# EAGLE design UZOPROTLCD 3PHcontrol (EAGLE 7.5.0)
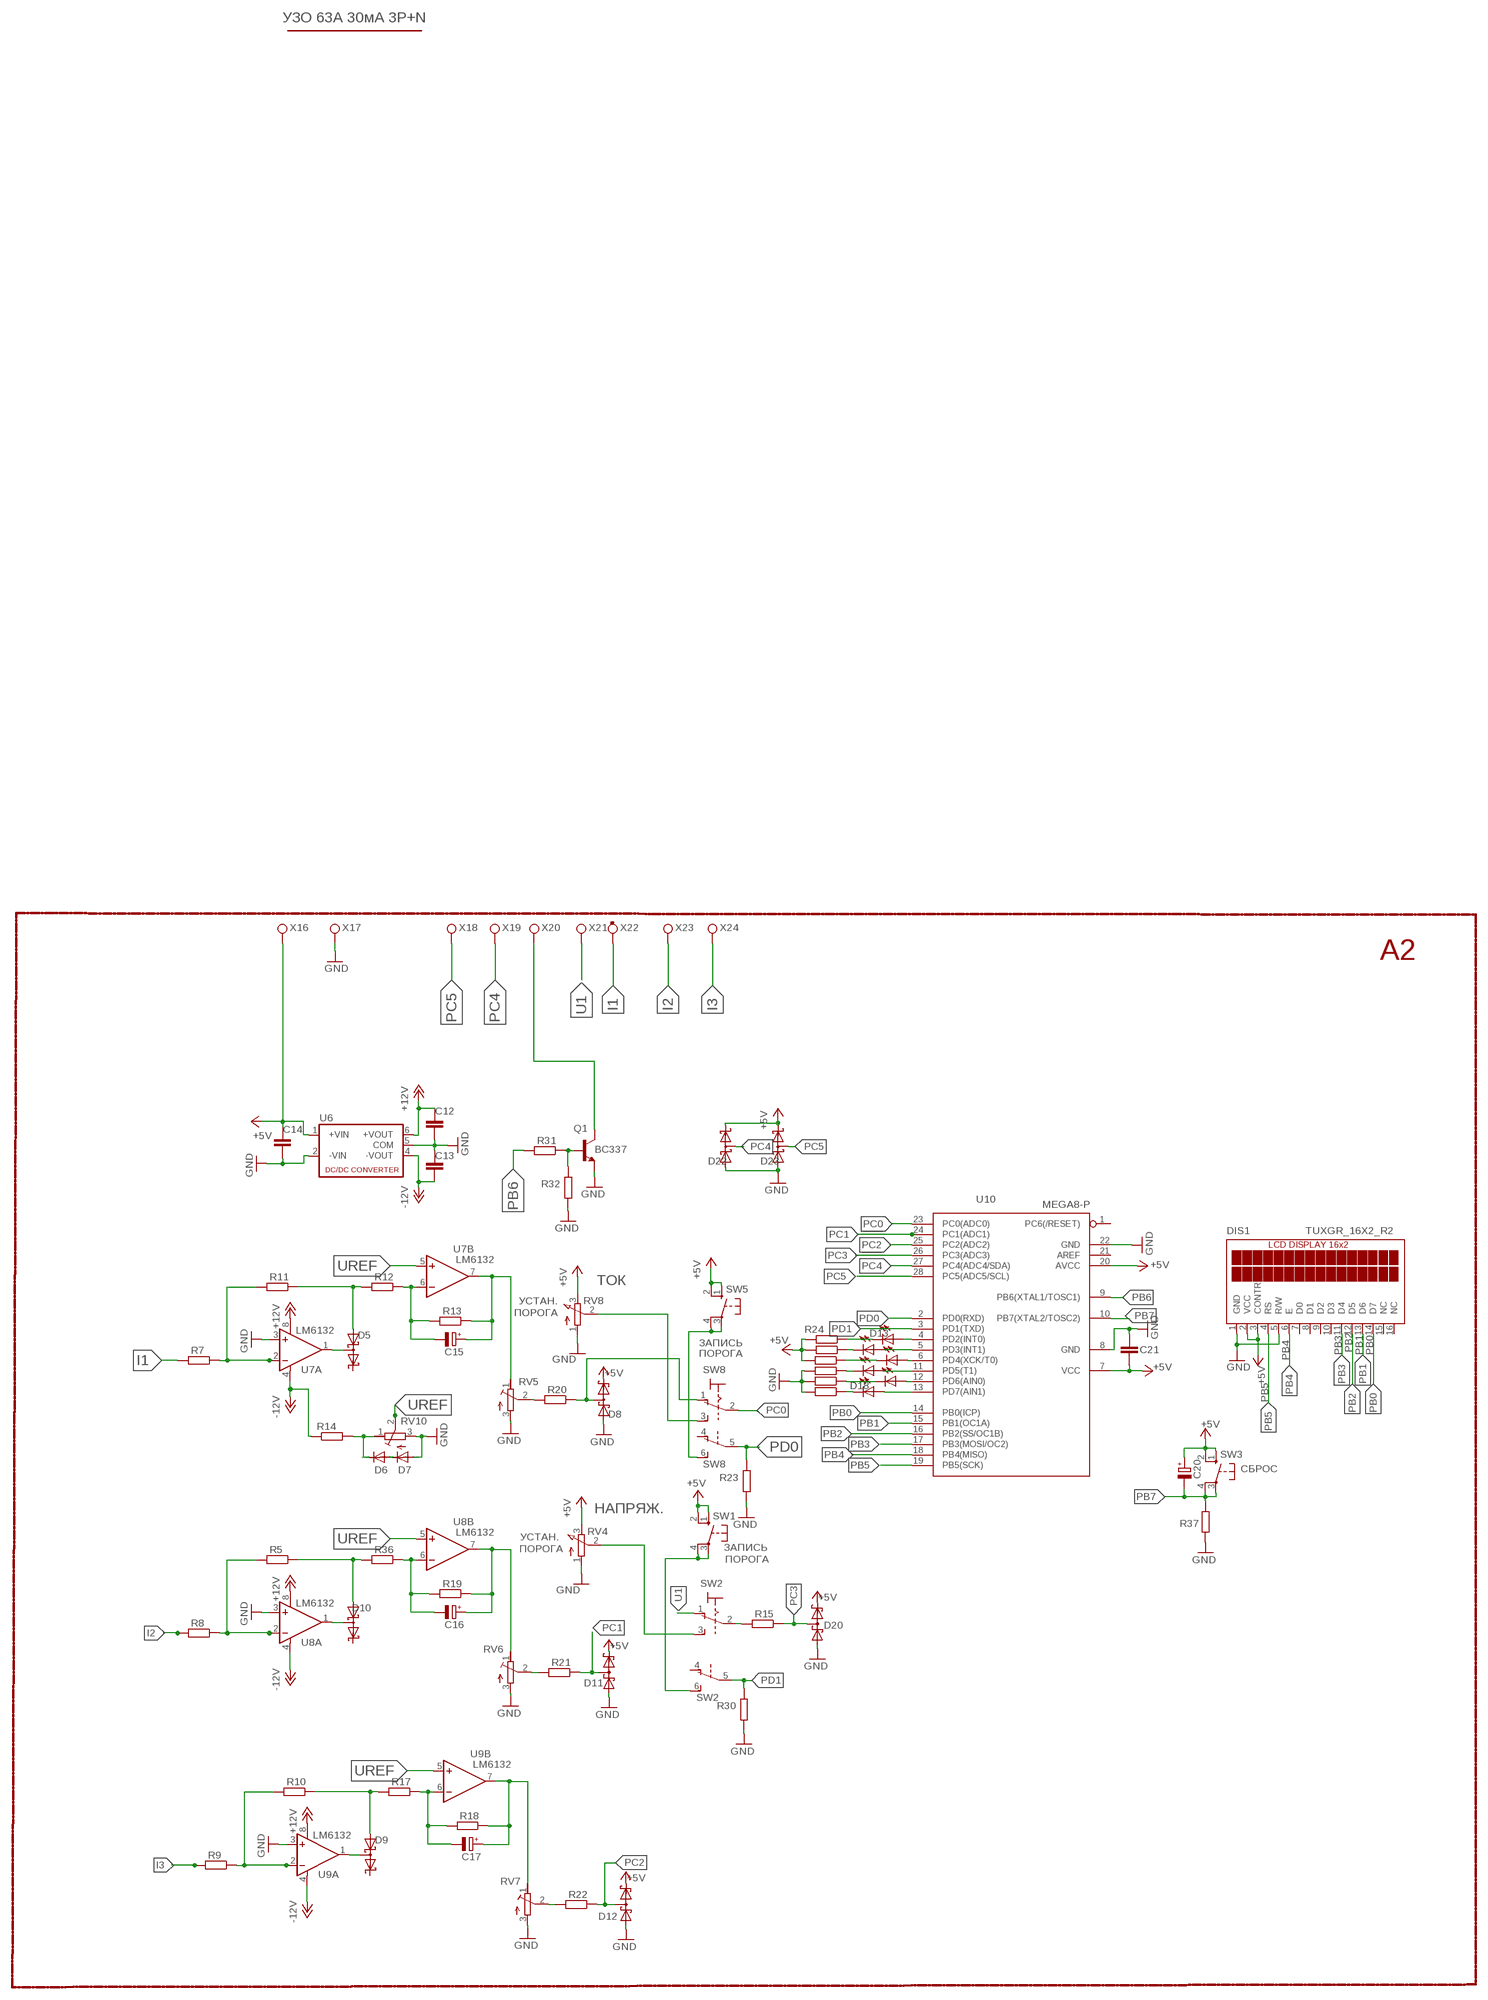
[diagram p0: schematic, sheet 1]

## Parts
C12  C-EUC1206  [C1206]
C13  C-EUC1206  [C1206]
C14  C-EUC1206  [C1206]
C15  CPOL-EUE2-4  [E2-4]
C16  CPOL-EUE2-4  [E2-4]
C17  CPOL-EUE2-4  [E2-4]
C20  CPOL-EUE2-5  [E2-5]
C21  C-EUC1206  [C1206]
D5  BAT54S  [SOT23]
D6  1N4148DO35-7  [DO35-7]
D7  1N4148DO35-7  [DO35-7]
D8  BAT54S  [SOT23]
D9  BAT54S  [SOT23]
D10  BAT54S  [SOT23]
D11  BAT54S  [SOT23]
D12  BAT54S  [SOT23]
D13  LED3MM  [LED3MM]
D14  LED3MM  [LED3MM]
D15  LED3MM  [LED3MM]
D16  LED3MM  [LED3MM]
D17  LED3MM  [LED3MM]
D18  LED3MM  [LED3MM]
D20  BAT54S  [SOT23]
D22  BAT54S  [SOT23]
D23  BAT54S  [SOT23]
DIS1  TUXGR_16X2_R2  [TUXGR_16X2_R2]
Q1  BC337  [TO92]
R5  R-EU_R1206  [R1206]
R7  R-EU_R1206  [R1206]
R8  R-EU_R1206  [R1206]
R9  R-EU_R1206  [R1206]
R10  R-EU_R1206  [R1206]
R11  R-EU_R1206  [R1206]
R12  R-EU_R1206  [R1206]
R13  R-EU_R1206  [R1206]
R14  R-EU_R1206  [R1206]
R15  R-EU_R1206  [R1206]
R17  R-EU_R1206  [R1206]
R18  R-EU_R1206  [R1206]
R19  R-EU_R1206  [R1206]
R20  R-EU_R1206  [R1206]
R21  R-EU_R1206  [R1206]
R22  R-EU_R1206  [R1206]
R23  R-EU_R1206  [R1206]
R24  R-EU_R1206  [R1206]
R25  R-EU_R1206  [R1206]
R26  R-EU_R1206  [R1206]
R27  R-EU_R1206  [R1206]
R28  R-EU_R1206  [R1206]
R29  R-EU_R1206  [R1206]
R30  R-EU_R1206  [R1206]
R31  R-EU_R1206  [R1206]
R32  R-EU_R1206  [R1206]
R36  R-EU_R1206  [R1206]
R37  R-EU_R1206  [R1206]
RV4  PTV09A  PV09A  [PTV09]
RV5  R-TRIMM-3386-F  [R-TRIMM-3386F]
RV6  R-TRIMM-3386-F  [R-TRIMM-3386F]
RV7  R-TRIMM-3386-F  [R-TRIMM-3386F]
RV8  PTV09A  PV09A  [PTV09]
RV10  R-TRIMM-3386-F  [R-TRIMM-3386F]
SW1  SPST Push Button  10-XX  [B3F-10XX]
SW2  320-938  [320-938]
SW3  SPST Push Button  10-XX  [B3F-10XX]
SW5  SPST Push Button  10-XX  [B3F-10XX]
SW8  320-938  [320-938]
U6  NMA  [NMA]
U7  LM6132  OPA2134P  [DIL08]
U8  LM6132  OPA2134P  [DIL08]
U9  LM6132  OPA2134P  [DIL08]
U10  MEGA8-P  [DIL28-3]
X16  TPPAD1-17  [P1-17]
X17  TPPAD1-17  [P1-17]
X18  TPPAD1-17  [P1-17]
X19  TPPAD1-17  [P1-17]
X20  TPPAD1-17  [P1-17]
X21  TPPAD1-17  [P1-17]
X22  TPPAD1-17  [P1-17]
X23  TPPAD1-17  [P1-17]
X24  TPPAD1-17  [P1-17]

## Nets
+5V: C14.1 C20.+ C21.2 D8.2(C2) D11.2(C2) D12.2(C2) D20.2(C2) D22.2(C2) D23.2(C2) DIS1.2(VCC) DIS1.3(CONTR) R24.2 R25.2 R26.2 RV4.3(E) RV8.3(E) SW1.1(S) SW1.2(S1) SW3.1(S) SW3.2(S1) SW5.1(S) SW5.2(S1) U6.1(+VIN) U10.7(VCC) U10.20(AVCC) X16.TP
+12V: C12.1 U6.6(+VOUT) U7.8(A:V+) U8.8(A:V+) U9.8(A:V+)
-12V: C13.2 R14.1 U6.4(-VOUT) U7.4(A:V-) U8.4(A:V-) U9.4(A:V-)
GND: C12.2 C13.1 C14.2 C21.1 D7.A D8.1(A1) D11.1(A1) D12.1(A1) D20.1(A1) D22.1(A1) D23.1(A1) DIS1.1(GND) DIS1.5(R/W) Q1.1(E) R23.2 R27.2 R28.2 R29.2 R30.2 R32.2 R37.2 RV4.1(A) RV5.3(E) RV6.3(E) RV7.3(E) RV8.1(A) RV10.3(E) U6.2(-VIN) U6.5(COM) U7.3(A:+IN) U8.3(A:+IN) U9.3(A:+IN) U10.8(GND) U10.22(GND) X17.TP
I1: R7.2 X22.TP
I2: R8.2 X23.TP
I3: R9.2 X24.TP
N$40: Q1.2(B) R31.1 R32.1
N$41: R7.1 R11.2 U7.2(A:-IN)
N$42: Q1.3(C) X20.TP
N$43: D6.C R14.2 RV10.1(A)
N$44: D6.A D7.C
N$45: D5.1(A1) R11.1 R12.2
N$46: D5.3(C1A2) U7.1(A:OUT)
N$47: C15.- R12.1 R13.2 U7.6(B:-IN)
N$48: C15.+ R13.1 RV5.1(A) U7.7(B:OUT)
N$49: R20.2 RV5.2(S)
N$50: RV8.2(S) SW8.3(1:S)
N$51: SW5.3(P) SW5.4(P1) SW8.6(B:S)
N$52: D8.3(C1A2) R20.1 SW8.1(1:O)
N$53: R9.1 R10.2 U9.2(A:-IN)
N$54: R5.2 R8.1 U8.2(A:-IN)
N$55: D10.1(A1) R5.1 R36.2
N$56: D10.3(C1A2) U8.1(A:OUT)
N$57: C16.- R19.2 R36.1 U8.6(B:-IN)
N$58: C16.+ R19.1 RV6.1(A) U8.7(B:OUT)
N$59: R21.2 RV6.2(S)
N$60: D9.1(A1) R10.1 R17.2
N$61: D9.3(C1A2) U9.1(A:OUT)
N$62: C17.- R17.1 R18.2 U9.6(B:-IN)
N$63: C17.+ R18.1 RV7.1(A) U9.7(B:OUT)
N$64: R22.2 RV7.2(S)
N$65: RV4.2(S) SW2.3(1:S)
N$66: SW1.3(P) SW1.4(P1) SW2.6(B:S)
N$67: R15.2 SW2.2(1:P)
N$68: D13.A U10.4(PD2(INT0))
N$69: D13.K(C) R24.1
N$70: D14.A U10.5(PD3(INT1))
N$71: D14.K(C) R25.1
N$72: D15.K(C) R26.1
N$74: D16.K(C) R27.1
N$75: D17.K(C) R28.1
N$76: D18.K(C) R29.1
N$77: D15.A U10.6(PD4(XCK/T0))
N$78: D16.A U10.11(PD5(T1))
N$79: D17.A U10.12(PD6(AIN0))
N$80: D18.A U10.13(PD7(AIN1))
PB0: DIS1.14(D7) U10.14(PB0(ICP))
PB1: DIS1.13(D6) U10.15(PB1(OC1A))
PB2: DIS1.12(D5) U10.16(PB2(SS/OC1B))
PB3: DIS1.11(D4) U10.17(PB3(MOSI/OC2))
PB4: DIS1.6(E) U10.18(PB4(MISO))
PB5: DIS1.4(RS) U10.19(PB5(SCK))
PB6: R31.2 U10.9(PB6(XTAL1/TOSC1))
PB7: C20.- R37.1 SW3.3(P) SW3.4(P1) U10.10(PB7(XTAL2/TOSC2))
PC0: SW8.2(1:P) U10.23(PC0(ADC0))
PC1: D11.3(C1A2) R21.1 U10.24(PC1(ADC1))
PC2: D12.3(C1A2) R22.1 U10.25(PC2(ADC2))
PC3: D20.3(C1A2) R15.1 U10.26(PC3(ADC3))
PC4: D22.3(C1A2) U10.27(PC4(ADC4/SDA)) X19.TP
PC5: D23.3(C1A2) U10.28(PC5(ADC5/SCL)) X18.TP
PD0: R23.1 SW8.5(B:P) U10.2(PD0(RXD))
PD1: R30.1 SW2.5(B:P) U10.3(PD1(TXD))
U1: SW2.1(1:O) X21.TP
UREF: RV10.2(S) U7.5(B:+IN) U8.5(B:+IN) U9.5(B:+IN)
Unconnected: D5.2(C2) D9.2(C2) D10.2(C2) DIS1.7(D0) DIS1.8(D1) DIS1.9(D2) DIS1.10(D3) DIS1.15(NC) DIS1.16(NC) SW2.4(B:O) SW8.4(B:O) U10.1(PC6(/RESET)) U10.21(AREF)

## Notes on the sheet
- УЗО 63А 30мА 3Р+N
- A2
- ТОК
- УСТАН.
- ПОРОГА
- ЗАПИСЬ
- ПОРОГА
- СБРОС
- НАПРЯЖ.
- УСТАН.
- ПОРОГА | ЗАПИСЬ
- ПОРОГА

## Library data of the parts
C12-C14 C21 = rcl:C-EU: CAPACITOR, European symbol
C15-C17 C20 = rcl:CPOL-EU: POLARIZED CAPACITOR, European symbol
D5 D8-D12 D20 D22 D23 = diode:BAT54S: Schottky Diodes Pin connection corrected 2011-05-04 Source: Fairchild .. BAT54.pdf
D6 D7 = diode:1N4148: DIODE
D13-D18 = led:LED: LED
DIS1 = display-lcd:TUXGR_16X2_R2: Tuxgraphics LCD display 16x2 characters reflective, without background light Source: tuxgr_12x2_r2.pdf; OC_FARNELL: unknown; OC_NEWARK: unknown
Q1 = transistor:BC337: NPN TRANSISTOR
R5 R7-R15 R17-R32 R36 R37 = rcl:R-EU_: RESISTOR, European symbol
RV4 RV8 = pot:PV09A
RV5-RV7 RV10 = rcl:R-TRIMM-3386-F
SW1 SW3 SW5 = switch-omron:10-XX: OMRON SWITCH; MPN: B3F-1000; OC_FARNELL: 176432; OC_NEWARK: 36M3542
SW2 SW8 = switch:320-938: TOGGLE SWITCH distributor RS Components
U6 = dc-dc-converter:NMA: DC-DC CONVERTER; MF: C & D TECHNOLOGIES, INC; MPN: NMA0515SC; OC_FARNELL: 1021434; OC_NEWARK: 61K3064
U7-U9 = burr-brown:OPA2134: Operational Amplifier; MF: TEXAS INSTRUMENTS; MPN: OPA2134PA; OC_FARNELL: 1097574; OC_NEWARK: 74K3897
U10 = atmel:MEGA8-P: MICROCONTROLLER 8 Kbytes FLASH, 1 kbytes SRAM, 512 bytes EEPROM, USART, 4-channel 10 bit ADC, 2-channel 8 bit ADC Pin compatible with Atmega48, ATMega88, ATMega168 Source: avr.lbr; OC_FARNELL: unknown; OC_NEWARK: unknown
X16-X24 = testpad:TP: Test pad

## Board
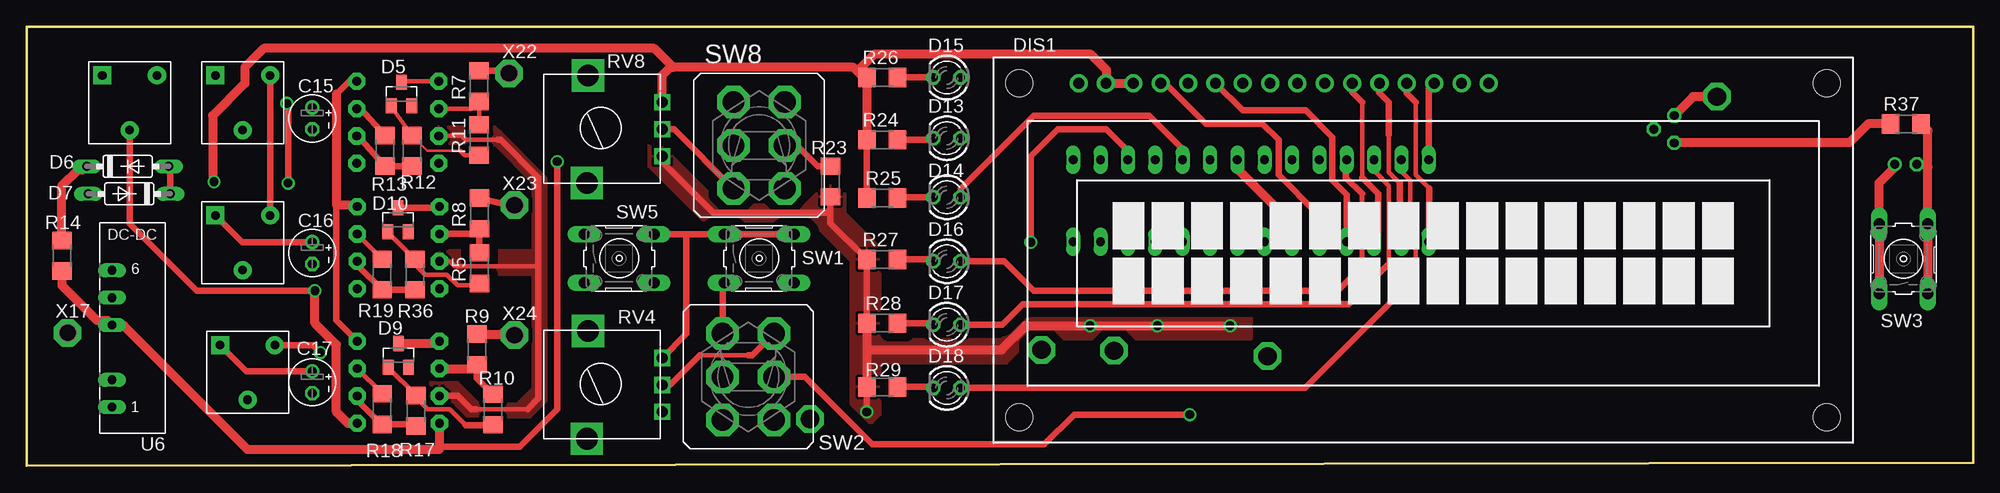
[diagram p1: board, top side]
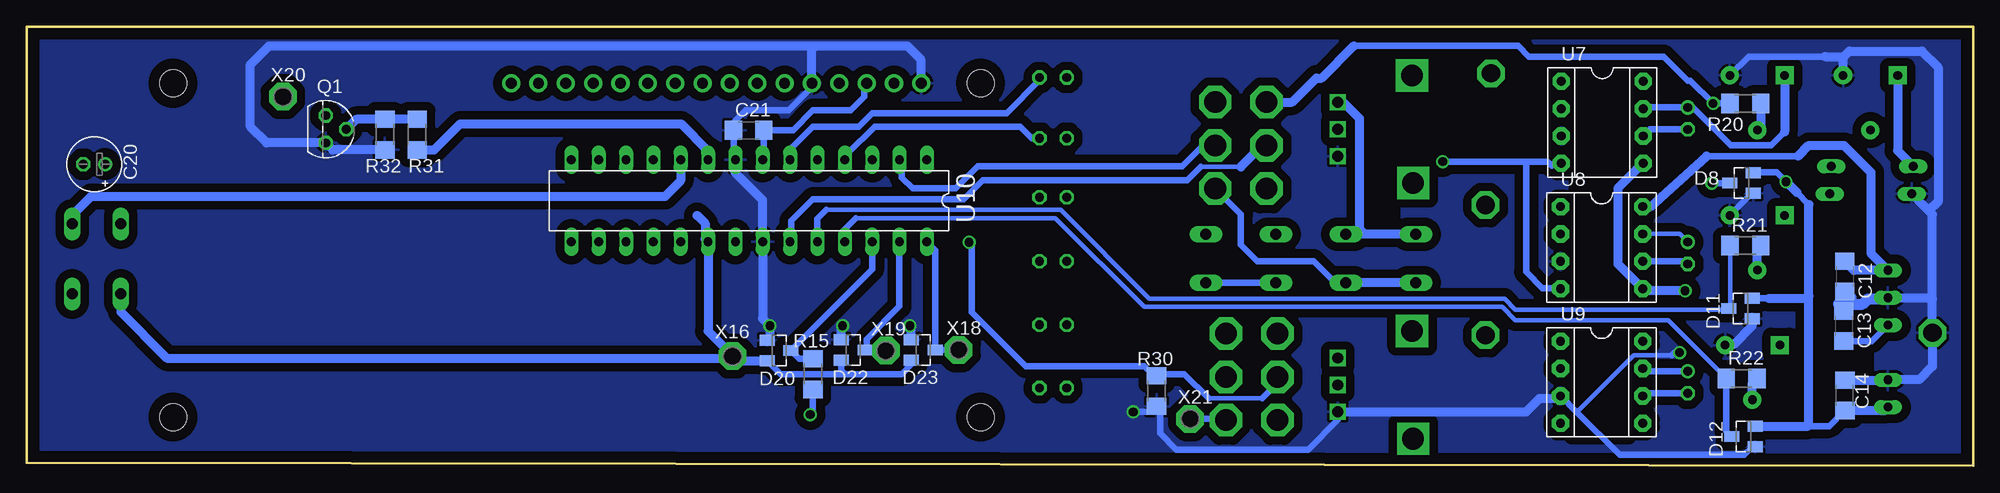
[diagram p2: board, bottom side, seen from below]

Size 180.75 x 40.75 mm. Coordinates in mm from the lower left corner, seen from the top.
Outline: 0,0 180.75,0.25 180.75,40.75 0,40.75 0,0
Copper layers (1*16): Top 0.035mm / dielectric 1.5mm / Bottom 0.035mm
Design rules "default": minimum track width 10mil, minimum drill 24mil, track to track 8mil, track to pad 8mil, pad to pad 8mil, via to via 8mil, smd to smd 8mil, copper to edge 40mil, drill to drill 8mil, minimum pad ring 10mil, minimum via ring 8mil, stop-mask expansion 4mil, vias tented up to drill 0mil, thermal gap 10mil
bRestrict: area 10,4.8 to 14.5,24.5; area 10.5,23.8 to 12.5,24; area 31.8,15.2 to 36.8,37; area 32,2.8 to 37.2,12.8; area 39.2,29.2 to 55.5,37; area 54,23 to 55.8,28.8

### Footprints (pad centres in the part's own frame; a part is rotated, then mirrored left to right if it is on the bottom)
C1206 = smd 1.6 x 1.8: 1 -1.4,0; 2 1.4,0
E2-4 = drill 0.813 pad 1.27: + -1.016,0 | drill 0.813 pad 1.27 octagon: - 1.016,0
E2-5 = drill 0.813 pad 1.27: + -1.016,0 | drill 0.813 pad 1.27 octagon: - 1.016,0
SOT23 = smd 1 x 1.4: 1 -0.95,-1.1; 2 0.95,-1.1; 3 0,1.1
DO35-7 = drill 0.813 long: A 3.81,0; C -3.81,0
LED3MM = drill 0.813 octagon: A -1.27,0; K 1.27,0
TUXGR_16X2_R2 = drill 1 pad 1.676: 1 -32,15.5; 2 -29.46,15.5; 3 -26.92,15.5; 4 -24.38,15.5; 5 -21.84,15.5; 6 -19.3,15.5; 7 -16.76,15.5; 8 -14.22,15.5; 9 -11.68,15.5; 10 -9.14,15.5; 11 -6.6,15.5; 12 -4.06,15.5; 13 -1.52,15.5; 14 1.02,15.5; 15 3.56,15.5; 16 6.1,15.5 | hole 2.5: -37.5,-15.5; 37.5,-15.5; -37.5,15.5; 37.5,15.5
TO92 = drill 0.813 octagon: 1 1.27,0; 2 0,1.905; 3 -1.27,0
R1206 = smd 1.6 x 1.803: 1 -1.422,0; 2 1.422,0
PTV09 = drill 1 square: 1 -2.5,0; 2 0,0; 3 2.5,0 | drill 2 square: P$4 -5,7; P$5 5,6.9
R-TRIMM-3386F = drill 0.8 pad 1.676 square: 1 0,0 | drill 0.8 pad 1.676: 2 5.08,2.54; 3 0,5.08
B3F-10XX = drill 1.016 long: 1 -3.251,2.261; 2 3.251,2.261; 3 -3.251,-2.261; 4 3.251,-2.261
320-938 = drill 2.007 octagon: 1 -2.388,4.013; 2 -2.388,0; 3 -2.388,-4.013; 4 2.388,4.013; 5 2.388,0; 6 2.388,-4.013
NMA = drill 0.813 long: 1 0,6.35; 2 0,3.81; 4 0,-1.27; 5 0,-3.81; 6 0,-6.35
DIL08 = drill 0.813 pad 1.6 octagon: 1 -3.81,-3.81; 2 -1.27,-3.81; 3 1.27,-3.81; 4 3.81,-3.81; 5 3.81,3.81; 6 1.27,3.81; 7 -1.27,3.81; 8 -3.81,3.81
DIL28-3 = drill 0.813 long: 1 -16.51,-3.81; 2 -13.97,-3.81; 3 -11.43,-3.81; 4 -8.89,-3.81; 5 -6.35,-3.81; 6 -3.81,-3.81; 7 -1.27,-3.81; 8 1.27,-3.81; 9 3.81,-3.81; 10 6.35,-3.81; 11 8.89,-3.81; 12 11.43,-3.81; 13 13.97,-3.81; 14 16.51,-3.81; 15 16.51,3.81; 16 13.97,3.81; 17 11.43,3.81; 18 8.89,3.81; 19 6.35,3.81; 20 3.81,3.81; 21 1.27,3.81; 22 -1.27,3.81; 23 -3.81,3.81; 24 -6.35,3.81; 25 -8.89,3.81; 26 -11.43,3.81; 27 -13.97,3.81; 28 -16.51,3.81
P1-17 = drill 1.702 pad 2.54 octagon: TP 0,0

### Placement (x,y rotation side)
C12  11.92,17.58 270 bottom
C13  12.01,12.97 270 bottom
C14  11.91,6.53 90 bottom
C15  26.5,32.25 270 top
C16  26.5,19.75 270 top
C17  26.5,7.75 270 top
C20  174.5,28 180 bottom
C21  113.72,31.15 0 bottom
D5  34.78,34.52 0 top
D6  9.36,27.8 0 top
D7  9.5,25.25 180 top
D8  21.5,26.25 90 bottom
D9  34.5,10.25 0 top
D10  34.47,22.84 0 top
D11  21.61,14.6 90 bottom
D12  21.33,2.72 90 bottom
D13  85.44,30.42 180 top
D14  85.44,24.93 180 top
D15  85.44,36.05 180 top
D16  85.44,18.98 180 top
D17  85.44,13.1 180 top
D18  85.44,7.22 180 top
D20  110.89,10.69 270 bottom
D22  104,10.75 270 bottom
D23  97.5,10.75 270 bottom
DIS1  129.68,20.02 0 top
Q1  153,31.25 270 bottom
R5  42.03,18.35 90 top
R7  42,35.25 90 top
R8  42.03,23.43 90 top
R9  41.79,10.8 90 top
R10  43.29,5.22 90 top
R11  42,30.25 90 top
R12  35.75,29.25 90 top
R13  33.25,29.25 270 top
R14  3.25,19.5 90 top
R15  107.75,8.5 270 bottom
R17  36.14,5.1 90 top
R18  33,5.25 270 top
R19  33,17.75 270 top
R20  21.15,33.64 0 bottom
R21  21.15,20.44 0 bottom
R22  21.49,8.11 0 bottom
R23  74.63,26.4 270 top
R24  79.44,30.27 180 top
R25  79.44,24.85 180 top
R26  79.44,36.07 180 top
R27  79.44,19.15 180 top
R28  79.44,13.23 180 top
R29  79.44,7.31 180 top
R30  75.84,6.94 270 bottom
R31  144.5,30.75 270 bottom
R32  147.5,30.75 270 bottom
R36  36.03,17.76 90 top
R37  174.5,31.75 180 top
RV4  59,7.5 90 top
RV5  17.5,36.25 270 top
RV6  17.5,23.25 270 top
RV7  17.95,11.2 270 top
RV8  59,31.25 90 top
RV10  7,36.25 270 top
SW1  68,19.25 0 top
SW2  67,8.25 180 top
SW3  174.29,19.21 90 top
SW5  55,19.25 0 top
SW8  68,29.75 0 top
U6  7.91,11.79 180 top
U7  34.44,31.89 270 bottom
U8  34.5,20.25 270 bottom
U9  34.5,7.75 270 bottom
U10  113.68,24.61 180 bottom
X16  115.22,10.17 0 bottom
X17  3.78,12.34 0 top
X18  94.22,10.76 0 bottom
X19  100.97,10.68 0 bottom
X20  156.97,34.27 0 bottom
X21  72.72,4.35 0 bottom
X22  44.78,36.44 0 top
X23  45.28,24.2 0 top
X24  45.28,12.12 0 top

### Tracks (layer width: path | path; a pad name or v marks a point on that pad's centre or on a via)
+5V  (via drill 0.8)
  Top 0.61: R25.2 R24.2 | SW5.2 61.25,21.51 | 61.25,21.51 SW1.1 SW1.2 | RV4.3 61.25,12.25 61.25,21.51
  Top 0.813: 77.12,36.62 77.68,36.07 R26.2 R24.2 | 77.12,36.62 76.75,37 60,37 59.88,37.12 | U10.7 112.41,27.59 117.25,22.75 117.25,21.04 U10.20 | C20.+ 173.48,27.73 172,26.25 172,22.49 SW3.2 SW3.1 | 77.12,36.62 78.75,38.25 98.75,38.25 100.25,36.75 100.25,35.55 DIS1.2 DIS1.3 | 59.88,37.12 58.25,38.75 22,38.75 20.25,37 20.25,35.5 17.25,32.5 17.25,26.5 v17.38,26.38 | RV8.3 59,36.25 59.88,37.12
  Bottom 0.61: U10.7 112.32,28.51 C21.2 109.6,31.15 107.75,33 104.25,33 103,34.25 103,35.28 DIS1.3 | D23.2 98.6,9.4 99.5,8.5 104.75,8.5 | 104.75,8.5 110.75,8.5 | 110.75,8.5 D20.2 | D22.2 105.1,8.85 104.75,8.5 | 110.72,8.47 110.75,8.5 | D20.2 114.8,9.75 X16.TP | D11.2 18.95,15.55 | D12.2 13.37,3.67 C14.1 | 15.25,24.25 16.38,25.38 | v17.38,26.38 18.25,27.25 20.35,27.25 D8.2
  Bottom 0.813: D20.2 114.75,9.75 117.49,12.49 U10.20 117.75,21.06 117.75,22.5 118.5,23.25 | SW3.1 172.03,14.28 167.75,10 115.05,10 114.8,9.75 | RV8.3 58.5,33.75 57,32.25 57,22.01 56.5,21.51 | SW5.1 56.5,21.51 | 56.5,21.51 SW5.2 | C14.1 8.22,5.13 U6.1 | D12.2 15.33,3.67 15.25,3.75 15.25,15.75 | 18.95,15.55 15.45,15.55 15.25,15.75 | 15.25,15.75 15.25,24.25 | v17.38,26.38 16.38,25.38
+12V
  Top 0.61: U7.8 29.95,35.7 28.75,34.5 | 28.75,24.25 28.75,13.5 U9.8
  Top 0.813: 28.75,34.5 28.75,24.25 30.5,24.25 U8.8
  Bottom 0.61: 24.75,28.75 16.25,28.75
  Bottom 0.813: C12.1 11.08,18.14 U6.6 9.5,19.73 9.5,27.25 12,29.75 15.25,29.75 16.25,28.75 | U8.8 29.94,24.06 24.75,28.75
-12V  (via drill 0.8)
  Top 0.61: 38.31,1.75 45.75,1.75 49.25,5.25 v49.25,28.25
  Top 0.813: U9.4 38.31,1.75 38.31,1.56 38.25,1.5 20.5,1.5 9,13 7.97,13 U6.4 7.47,13.5 6.5,13.5 3.25,16.75 R14.1
  Bottom 0.61: U7.4 38.92,28.08 39.12,27.88 39.5,28.25 41.5,28.25 | 41.5,28.25 41.5,18 40,16.5 38.37,16.5 U8.4 | v49.25,28.25 41.5,28.25 | C13.2 9.4,11.57 U6.4
GND  (via drill 0.8)
  Top 0.406: U7.3 40.38,30.62 40.75,30.25 43.75,30.25 | 47.5,18.5 39.75,18.5 39.25,19 38.33,19 U8.3 | 46.5,5.25 41.75,5.25
  Top 0.61: R23.2 74.63,23.75 | 74.63,23.75 74.63,22.54 R27.2 R28.2 78.02,10.77 78,10.75 | RV8.1 59,28.25 63.75,23.5 74.38,23.5 74.63,23.75 | R29.2 78.02,5.02 v78,5 | 43.75,30.25 44,30.25 47.5,26.75 47.5,18.5 47.5,6.25 46.5,5.25 | 41.75,5.25 41.25,5.25 40,6.5 38.33,6.5 U9.3 | RV6.3 RV5.3 | v27.25,10.5 26.55,11.2 RV7.3
  Top 0.813: v111.75,13 v105,13 v98.75,13 92.75,13 90.5,10.75 78,10.75 | R28.2 R29.2 | R37.2 171,31.75 169.25,30 153.02,30 Q1.1
  Bottom 0.305: 11.75,14.5 11.5,14.5 11,15
  Bottom 0.406: 28,10.25 31.5,10.25 36.79,4.96
  Bottom 0.61: U10.8 115.12,28.59 C21.1 115,31.27 115,32 114,33 110,33 107.84,35.16 DIS1.5 | RV4.1 59,4.25 61.75,1.5 74,1.5 75.5,3 75.5,5.18 R30.2 76.36,5 v78,5 | RV10.3 12.08,36.33 | 13.75,38 20.83,38 RV5.3 | RV7.3 22.96,11.2 | D8.1 20.4,25.43 RV6.3 | D12.1 20.48,1.77 21.25,1 32.83,1 36.79,4.96 U9.3 | v27.25,10.5 27.75,10.5 28,10.25
  Bottom 0.813: D20.1 111.75,11.88 v111.75,13 112.41,13.66 U10.22 112.41,24.66 115,27.25 115,28.37 U10.8 | D22.1 105.1,12.9 v105,13 | D23.1 98.6,12.85 v98.75,13 | R32.2 152.35,29.33 Q1.1 158.48,29.98 160,31.5 160,37.25 158.25,39 107.5,39 | 107.5,39 99,39 97.75,37.75 97.75,35.59 DIS1.1 | DIS1.5 107.84,38.66 107.5,39 | RV4.1 41.5,5 40.25,6.25 38.54,6.25 U9.3 | 12.01,16.09 C12.2 11.34,15.6 | 12.14,14.5 C13.1 11.88,14.37 11.75,14.5 | 3.78,15.5 X17.TP 3.78,9.22 5,8 7.89,8 U6.2 7.96,7.93 C14.2 | 3.78,15.5 3.78,23.34 4.09,23.66 | 4.09,23.66 D7.A | U6.5 3.88,15.6 3.78,15.5 | D11.1 20.51,12.99 22.25,11.25 22.91,11.25 22.96,11.2 | 13.75,38 12,38 | 12,38 11.5,38.5 4.75,38.5 3.25,37 3.25,24.5 4.09,23.66 | 12.08,36.33 12.08,37.92 12,38
  Bottom 1.016: 11.34,15.6 11.9,15.6 12.5,15 11,15 10.25,15 9.75,15.5 8.01,15.5 U6.5
  pour Bottom (isolate 0.8): 1,39.75 180,39.5 180,1 1,1.25
  pour Top (isolate 0.406): 44,31 48.25,26.75 48.25,6 46.75,4.5 38.5,4.5 37.25,5.75 37.25,7.5 37.5,7.75 40,7.75 42,5.75 45.5,5.75 47,7.25 47,26.25 43.5,29.75 37.75,29.75 37.5,30 37.5,31.25 37.75,31.5 43.5,31.5
  pour Top (isolate 0.813): 58.25,30 58.75,30 64.5,24.25 72.25,24.25 74,26 75.25,26 76,25.25 76,23.5 79.25,20.25 79.25,4.75 78.5,4 77.5,4 76.75,4.75 76.5,5 76.5,19 73,22.5 63,22.5 57.75,27.75 57.75,29.75 58,30
  pour Top (isolate 0.813): 79,11.75 90.5,11.75 92.5,13.75 113.75,13.75 113.75,11.75 93.25,11.75 91,9.5 79,9.5
  pour Top (isolate 0.813): 37.5,20 47,20 47.25,20.25 47.25,18 47.5,17.75 38,17.75 37.25,18.5 37.25,19.75
I1
  Top 0.61: R7.2 44.55,36.67 X22.TP
I2
  Top 0.61: R8.2 45.18,24.1 X23.TP
I3
  Top 0.813: R9.2 45.18,12.22 X24.TP
N$40
  Bottom 0.813: R31.1 R32.1 150.17,32.17 Q1.2
N$41
  Top 0.406: R11.2 R7.1 41.33,33.16 U7.2
N$42
  Top 0.813: X20.TP 154.75,34.27 Q1.3
N$43
  Top 0.813: R14.2 3.25,26 4.75,27.5 5.25,27.5 D6.C
  Bottom 0.813: 5.35,28 D6.C 7,29.25 RV10.1
N$44
  Top 0.61: D7.C 13.31,27.66 D6.A
N$45
  Top 0.254: 40.25,29.25 37.17,29.25 R12.2
  Top 0.406: D5.1 33.83,33.34 R12.2 | R11.1 40.67,28.83 40.25,29.25
N$46
  Top 0.406: U7.1 34.86,35.7 D5.3
N$47
  Top 0.61: U7.6 30.71,30.62 R13.2 R12.1
  Bottom 0.61: C15.- 30.02,31.23 U7.6
N$48
  Top 0.61: U7.7 31.01,33.16 R13.1
  Bottom 0.61: U7.7 30.52,33.27 C15.+ 26.48,33.25 26,33.25 22.5,29.75 18.75,29.75 17.5,31
  Bottom 0.813: RV5.1 17.5,31
N$49
  Bottom 0.813: R20.2 19.73,31.48 RV5.2
N$50
  Top 0.61: RV8.2 60.1,31.25 SW8.3
N$51
  Bottom 0.61: SW5.4 59.24,16.99 61.25,19 66.5,19 68,20.5 68,23.35 SW8.6
  Bottom 0.813: SW5.3 SW5.4
N$52  (via drill 0.8)
  Top 0.61: v24.25,26.25 24.25,33.53 v24.14,33.64
  Bottom 0.61: 22.6,33.61 R20.1 23.5,33.64 v24.14,33.64 26.25,35.75 26.5,35.75 28.75,38 41.25,38 42.25,39 57.5,39 | D8.3 v24.25,26.25
  Bottom 0.813: SW8.1 63.24,33.76 61,36 60.5,36 57.5,39
N$53
  Top 0.61: R9.1 41.79,8.14 R10.2
  Top 0.813: U9.2 41.43,9.02 R9.1
N$54
  Top 0.61: R5.2 R8.1 41.77,21.52 U8.2
N$55
  Top 0.406: D10.1 33.52,21.69 R36.2 36.03,18.72 37,17.75 39,17.75 40,16.75 41.85,16.75 R5.1
N$56
  Top 0.61: D10.3 38.19,23.94 U8.1
N$57
  Top 0.61: R36.1 R19.2 30.69,18.64 U8.6
  Bottom 0.61: U8.6 26.75,18.98 C16.-
N$58
  Top 0.406: U8.7 30.69,21.48 R19.1
  Top 0.61: C16.+ 19.98,20.77 RV6.1
  Bottom 0.406: U8.7 27.25,21.52 C16.+
N$59
  Bottom 0.813: RV6.2 20.04,19.63 R21.2
N$60
  Top 0.406: D9.1 33.55,9.11 R17.2 36.14,6.36 37.25,5.25 39.25,5.25 40.75,3.75
  Top 0.61: 40.75,3.75 43.24,3.75 R10.1
N$61
  Top 0.813: D9.3 38.1,11.35 U9.1
N$62
  Top 0.61: R17.1 35.99,3.83 R18.2 32.92,3.83 31,5.75 31,6.17 U9.6
  Bottom 0.61: C17.- 30.44,6.73 U9.6
N$63
  Top 0.406: R18.1 33,6.71 U9.7
  Top 0.61: C17.+ 20.38,8.77 RV7.1
  Bottom 0.61: C17.+ 30.44,8.77 U9.7
N$64
  Bottom 0.813: RV7.2 20.49,7.69 R22.2
N$65
  Top 0.406: 62.5,10.25 67,10.25
  Top 0.61: RV4.2 59.75,7.5 62.5,10.25 | 67,10.25 67.37,10.25 SW2.3
N$66
  Top 0.61: SW2.6 64.61,16.85 SW1.3
  Bottom 0.61: SW1.3 SW1.4
N$67  (via drill 0.8)
  Top 0.61: v108,4.75 97.25,4.75 94.5,2 78.5,2 72.25,8.25 SW2.2
  Bottom 0.61: R15.2 107.75,5 v108,4.75
N$68
  Bottom 0.61: D13.A 87.42,30.42 88.5,31.5 102,31.5 104.5,29 104.5,28.71 U10.4
N$69
  Top 0.61: R24.1 84.02,30.27 D13.K
N$70
  Top 0.61: D14.A 86.71,25.71 93.5,32.5 104.25,32.5 107.5,29.25 107.5,28.59 U10.5
N$71
  Top 0.61: D14.K 80.94,24.93 R25.1
N$72
  Top 0.61: R26.1 84.15,36.07 D15.K
N$74
  Top 0.61: R27.1 84,19.15 D16.K
N$75
  Top 0.61: R28.1 84.04,13.23 D17.K
N$76
  Top 0.61: R29.1 84.08,7.31 D18.K
N$77
  Bottom 0.61: D15.A 86.71,35.79 89.75,32.75 102.25,32.75 103.5,31.5 107.75,31.5 110,29.25 110,28.55 U10.6
N$78
  Top 0.45: 124,18.5 124,25.25
  Top 0.61: D16.A 90.77,18.98 93.5,16.25 121.75,16.25 124,18.5 | 124,25.25 122.5,26.75 122.5,28.35 U10.11
N$79
  Top 0.406: 126.5,18.75 126.5,26 125.25,27.25 125.25,28.28 U10.12
  Top 0.61: D17.A 90.6,13.1 92.5,15 122.75,15 126.5,18.75
N$80
  Top 0.406: U10.13 127.65,27.35 128.5,26.5 128.5,22.5 129,22 129,17.5
  Top 0.61: D18.A 118.72,7.22 129,17.5
PB0
  Top 0.61: U10.14 130.19,35.01 DIS1.14
PB1
  Top 0.406: 129,33.75 129,27 130.25,25.75
  Top 0.61: DIS1.13 128.16,34.59 129,33.75 | 130.25,25.75 130.25,20.86 U10.15
PB2
  Top 0.406: 126.5,30.75 126.5,27.25 127.5,26.25
  Top 0.61: DIS1.12 125.62,34.63 126.5,33.75 126.5,30.75 | 127.5,26.25 127.5,20.95 U10.16
PB3
  Top 0.406: 124,33.75 124,26.75
  Top 0.61: DIS1.11 123.08,34.67 124,33.75 | U10.17 125.5,21.19 125.5,25.25 124,26.75
PB4
  Top 0.61: U10.18 122.57,25.18 121.25,26.5 121.25,30.5 118.75,33 112.9,33 DIS1.6
PB5
  Top 0.61: DIS1.4 105.73,35.52 109.5,31.75 114.75,31.75 116.25,30.25 116.25,27 119.75,23.5 119.75,21.08 U10.19
PB6
  Bottom 0.813: R31.2 142.92,29.33 140.5,31.75 120,31.75 117.5,29.25 U10.9
PB7
  Top 0.813: 176.55,27.75 SW3.4 SW3.3 | 176.55,27.75 176.55,31.12 R37.1 | C20.- 176.3,28 176.55,27.75
  Bottom 0.813: U10.10 120.03,26.47 121.5,25 174.8,25 176.55,23.25 SW3.4
PC0
  Bottom 0.4: 68,27.75 71.75,27.75
  Bottom 0.61: 71.75,27.75 73,26.5 92,26.5 93.75,24.75 107.75,24.75 109.75,22.75 109.75,20.92 U10.23
  Bottom 0.813: SW8.2 66,29.75 68,27.75
PC1
  Bottom 0.406: 106.5,23.75 84.75,23.75 76.5,15.5 43.5,15.5 42.5,14.5 22.81,14.5 D11.3 22.57,14.74 R21.1
  Bottom 0.61: U10.24 107.33,22.92 106.5,23.75
PC2
  Bottom 0.406: 103.75,23 85.25,23 77,14.75 43.75,14.75 42.5,13.5 28.3,13.5 R22.1
  Bottom 0.61: U10.25 104.79,21.96 103.75,23 | R22.1 22.91,3.2 D12.3
PC3
  Bottom 0.61: U10.26 102.25,18.23 D20.3 109.02,9.92 R15.1
PC4
  Bottom 0.61: U10.27 99.71,14.79 102.75,11.75 102.75,10.9 | 102.75,10.9 D22.3 | 102.75,10.9 101.19,10.9 X19.TP
PC5
  Bottom 0.61: U10.28 96.4,20.03 D23.3 X18.TP
PD0
  Top 0.61: R23.1 73.43,27.82 71.5,29.75 SW8.5
  Bottom 0.61: U10.2 99.5,28.21 99.5,26.75 98.5,25.75 94.5,25.75 92.43,27.82 73.43,27.82 71.5,29.75 SW8.5
PD1  (via drill 0.8)
  Top 0.61: v93.25,20.75 93.25,28.75 95.75,31.25 100.25,31.25 102.25,29.25 U10.3
  Bottom 0.406: 66,6.25 71,6.25
  Bottom 0.61: v93.25,20.75 93,20.5 93,14.25 88,9.25 77,9.25 76.11,8.36 R30.1 75.7,8.5 73.25,8.5 71,6.25 | SW2.5 64.61,7.64 66,6.25
U1
  Bottom 0.61: X21.TP 69.5,4.35 SW2.1
UREF  (via drill 0.8)
  Top 0.61: RV10.2 9.54,22.46 15.75,16.25 v26.75,16.25
  Top 0.813: U9.5 29.81,3.94 28.75,5 28.75,11.25 26.75,13.25 v26.75,16.25
  Bottom 0.813: U7.5 30.67,28.08 33,25.75 33,18.75 U8.5 30.5,16.25 v26.75,16.25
